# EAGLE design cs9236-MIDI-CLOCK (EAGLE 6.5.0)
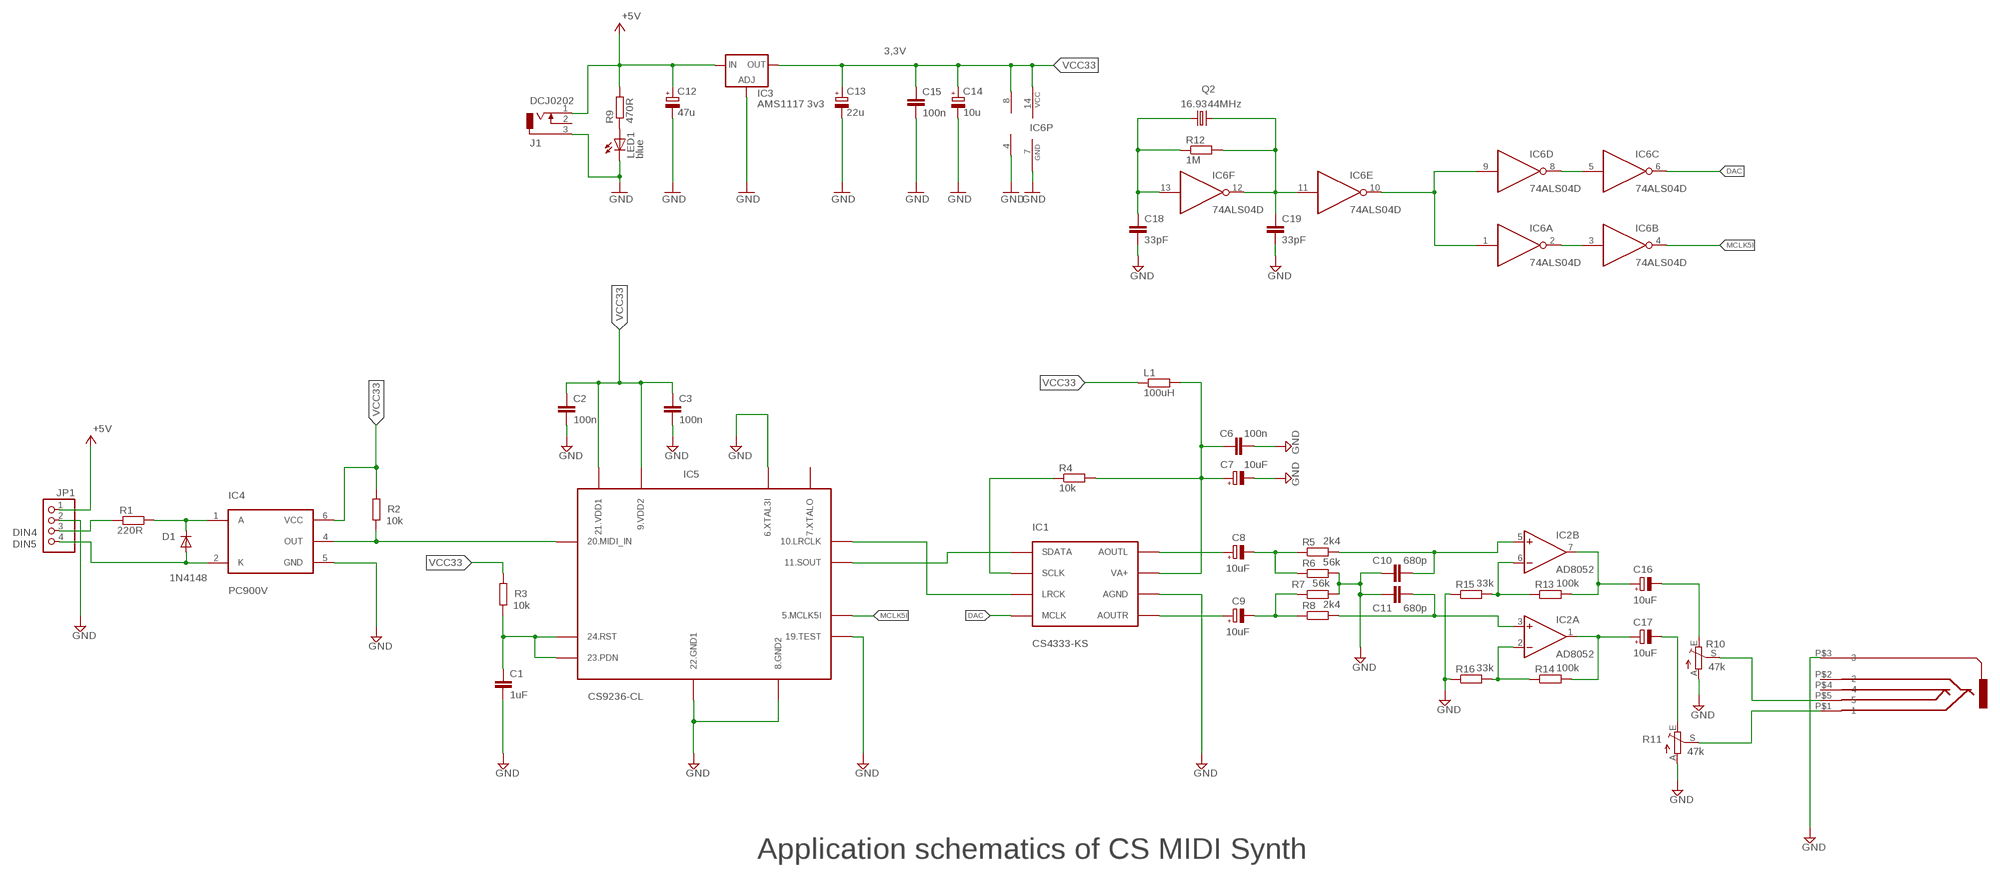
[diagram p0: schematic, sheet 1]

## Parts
C1  1uF  C-EUC0805  [C0805]
C2  100n  C-EUC0805  [C0805]
C3  100n  C-EUC0805  [C0805]
C6  100n  C-EUC0805  [C0805]
C7  10uF  CPOL-EUSMCC  [SMC_C]
C8  10uF  CPOL-EUSMCC  [SMC_C]
C9  10uF  CPOL-EUSMCC  [SMC_C]
C10  680p  C-EUC0805  [C0805]
C11  680p  C-EUC0805  [C0805]
C12  47u  CPOL-EUSMCD  [SMC_D]
C13  22u  CPOL-EUSMCD  [SMC_D]
C14  10u  CPOL-EUSMCB  [SMC_B]
C15  100n  C-EUC0805  [C0805]
C16  10uF  CPOL-EUSMCC  [SMC_C]
C17  10uF  CPOL-EUSMCC  [SMC_C]
C18  33pF  C-EUC0805  [C0805]
C19  33pF  C-EUC0805  [C0805]
D1  1N4148  1N4148DO35-7  [DO35-7]
IC1  CS4333-KS  [SO8]
IC2  AD8052  LM1458D  [SO08]
IC3  AMS1117 3v3  LD117AS33TR  [SOT223]
IC4  PC900V  [DIP6STD]
IC5  CS9236-CL  [PLCC28]
IC6  74ALS04D  [SO14]
J1  DCJ0202  [DCJ0202]
JP1  PINHD-1X4  [1X04]
L1  100uH  R-EU_0207/10  [0207/10]
LED1  blue  LEDSML0805  [SML0805]
Q2  16.9344MHz  CRYSTALHC49UP  [HC49UP]
R1  220R  R-EU_R0805  [R0805]
R2  10k  R-EU_R0805  [R0805]
R3  10k  R-EU_R0805  [R0805]
R4  10k  R-EU_R0805  [R0805]
R5  2k4  R-EU_R0805  [R0805]
R6  56k  R-EU_R0805  [R0805]
R7  56k  R-EU_R0805  [R0805]
R8  2k4  R-EU_R0805  [R0805]
R9  470R  R-EU_R0805  [R0805]
R10  47k  TRIM_EU-CT6  [CT6]
R11  47k  TRIM_EU-CT6  [CT6]
R12  1M  R-EU_R0805  [R0805]
R13  100k  R-EU_R0805  [R0805]
R14  100k  R-EU_R0805  [R0805]
R15  33k  R-EU_R0805  [R0805]
R16  33k  R-EU_R0805  [R0805]
U$3  JACK3.5  [JACK3.5]

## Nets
+5V: C12.+ IC3.3(IN) J1.1 JP1.1 R9.2
DAC: IC1.4(MCLK) IC6.6(C:O)
GND: C1.2 C2.2 C3.2 C6.2 C7.- C10.1 C11.1 C12.- C13.- C14.- C15.2 C18.2 C19.2 IC1.6(AGND) IC2.4(P:V-) IC3.1(ADJ) IC4.5(GND) IC5.6(6.XTAL3I) IC5.8(8.GND2) IC5.19(19.TEST) IC5.22(22.GND1) IC6.7(P:GND) J1.3 JP1.2 LED1.C R6.2 R7.2 R10.A R11.A R15.1 R16.1 U$3.P$3
MCLK5I: IC5.5(5.MCLK5I) IC6.4(B:O)
N$1: IC2.6(B:-IN) R13.1 R15.2
N$2: IC1.3(LRCK) IC5.10(10.LRCLK)
N$3: IC1.1(SDATA) IC5.11(11.SOUT)
N$4: C1.1 IC5.23(23.PDN) IC5.24(24.RST) R3.1
N$5: D1.C IC4.1(A) R1.1
N$6: IC4.4(OUT) IC5.20(20.MIDI_IN) R2.1
N$7: C9.+ IC1.5(AOUTR)
N$8: C8.+ IC1.8(AOUTL)
N$9: C6.1 C7.+ IC1.7(VA+) L1.2 R4.2
N$10: IC1.2(SCLK) R4.1
N$11: C8.- R5.1 R6.1
N$12: C9.- R7.1 R8.1
N$13: D1.A IC4.2(K) JP1.4
N$14: C18.1 IC6.13(F:I) Q2.1 R12.1
N$15: C11.2 IC2.3(A:+IN) R8.2
N$16: C10.2 IC2.5(B:+IN) R5.2
N$17: IC2.2(A:-IN) R14.1 R16.2
N$18: LED1.A R9.1
N$19: C16.+ IC2.7(B:OUT) R13.2
N$20: C17.+ IC2.1(A:OUT) R14.2
N$21: C16.- R10.E
N$22: C17.- R11.E
N$23: JP1.3 R1.2
N$24: R10.S U$3.P$5
N$25: R11.S U$3.P$1
N$26: C19.1 IC6.11(E:I) IC6.12(F:O) Q2.2 R12.2
N$27: IC6.1(A:I) IC6.9(D:I) IC6.10(E:O)
N$28: IC6.2(A:O) IC6.3(B:I)
N$29: IC6.5(C:I) IC6.8(D:O)
VCC33: C2.1 C3.1 C13.+ C14.+ C15.1 IC2.8(P:V+) IC3.4(OUT) IC4.6(VCC) IC5.9(9.VDD2) IC5.21(21.VDD1) IC6.14(P:VCC) L1.1 R2.2 R3.2
Unconnected: IC5.7(7.XTALO) J1.2 U$3.P$2 U$3.P$4

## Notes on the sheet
- 3,3V
- DIN4
- DIN5
- Application schematics of CS MIDI Synth

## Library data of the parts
C1-C3 C6 C10 C11 C15 C18 C19 = rcl:C-EU: CAPACITOR, European symbol
C7-C9 C12-C14 C16 C17 = rcl:CPOL-EU: POLARIZED CAPACITOR, European symbol
D1 = diode:1N4148: DIODE
IC1 = crystal-midi:CS4333-KS
IC2 = linear:*1458: OP AMP
IC3 = v-reg:LD117A?*: Low drop fixed and adjustable positive voltage regulators 1 A Source: http://www.st.com/stonline/products/literature/ds/7194/ld1117axx.pdf
IC4 = pc900:PC900V
IC5 = crystal-midi:CS9236-CL
IC6 = 74xx-us:74*04: Hex INVERTER
J1 = con-jack:DCJ0202: DC POWER JACK Source: DCJ0202.pdf; OC_FARNELL: unknown; OC_NEWARK: unknown
JP1 = pinhead:PINHD-1X4: PIN HEADER
L1 R1-R9 R12-R16 = rcl:R-EU_: RESISTOR, European symbol
LED1 = led:LED: LED
Q2 = crystal:CRYSTAL: CRYSTAL; OC_FARNELL: unknown; OC_NEWARK: unknown
R10 R11 = pot:TRIM_EU-: POTENTIOMETER
U$3 = CART-Z7:JACK3.5

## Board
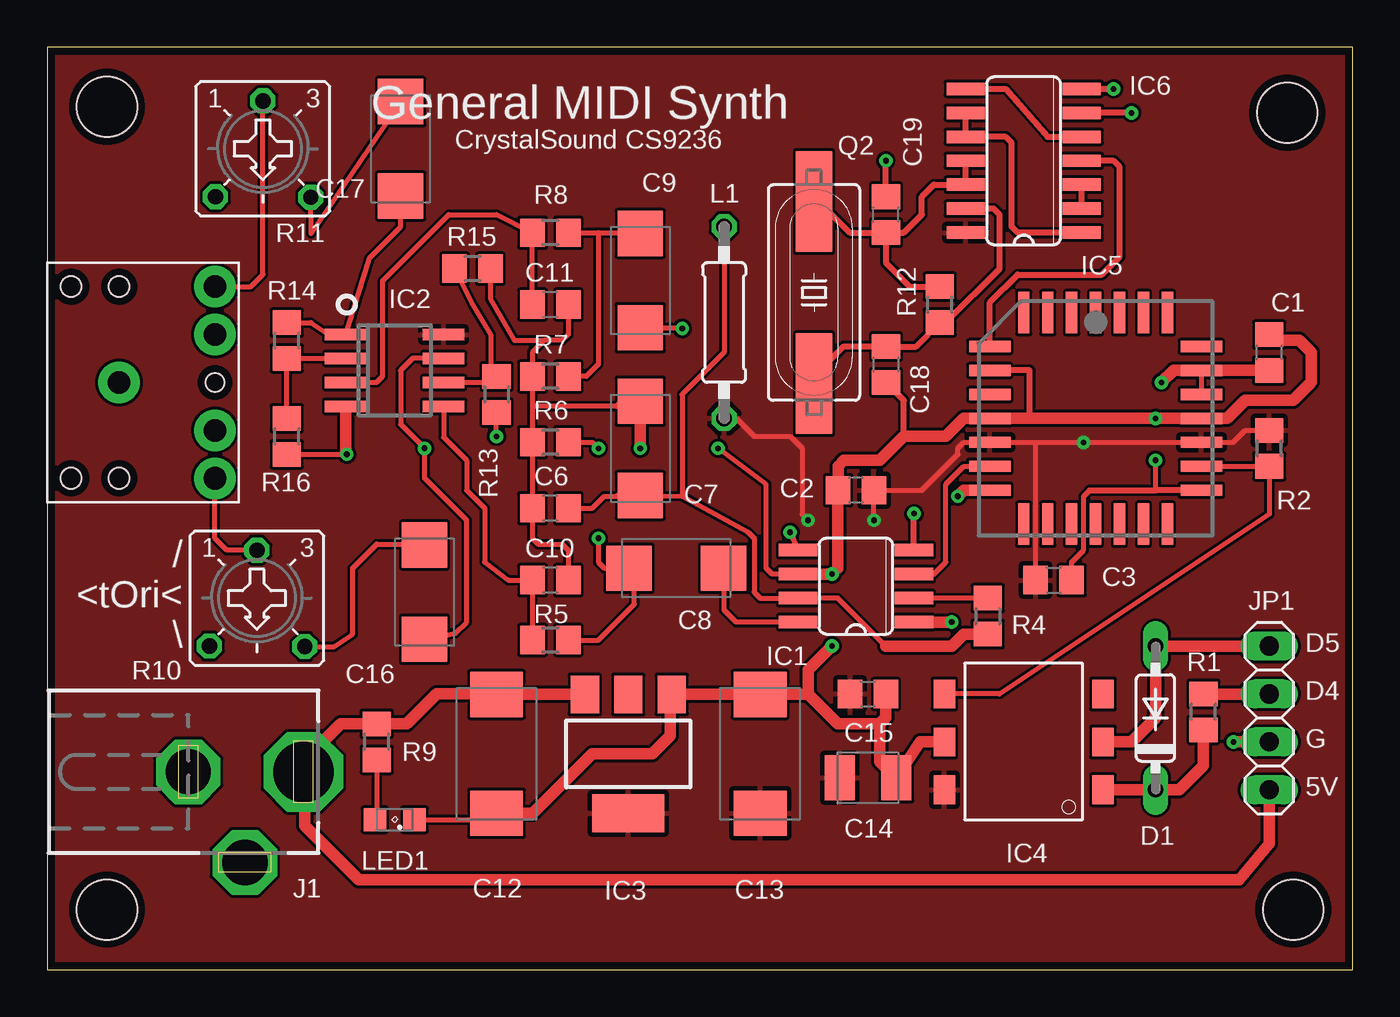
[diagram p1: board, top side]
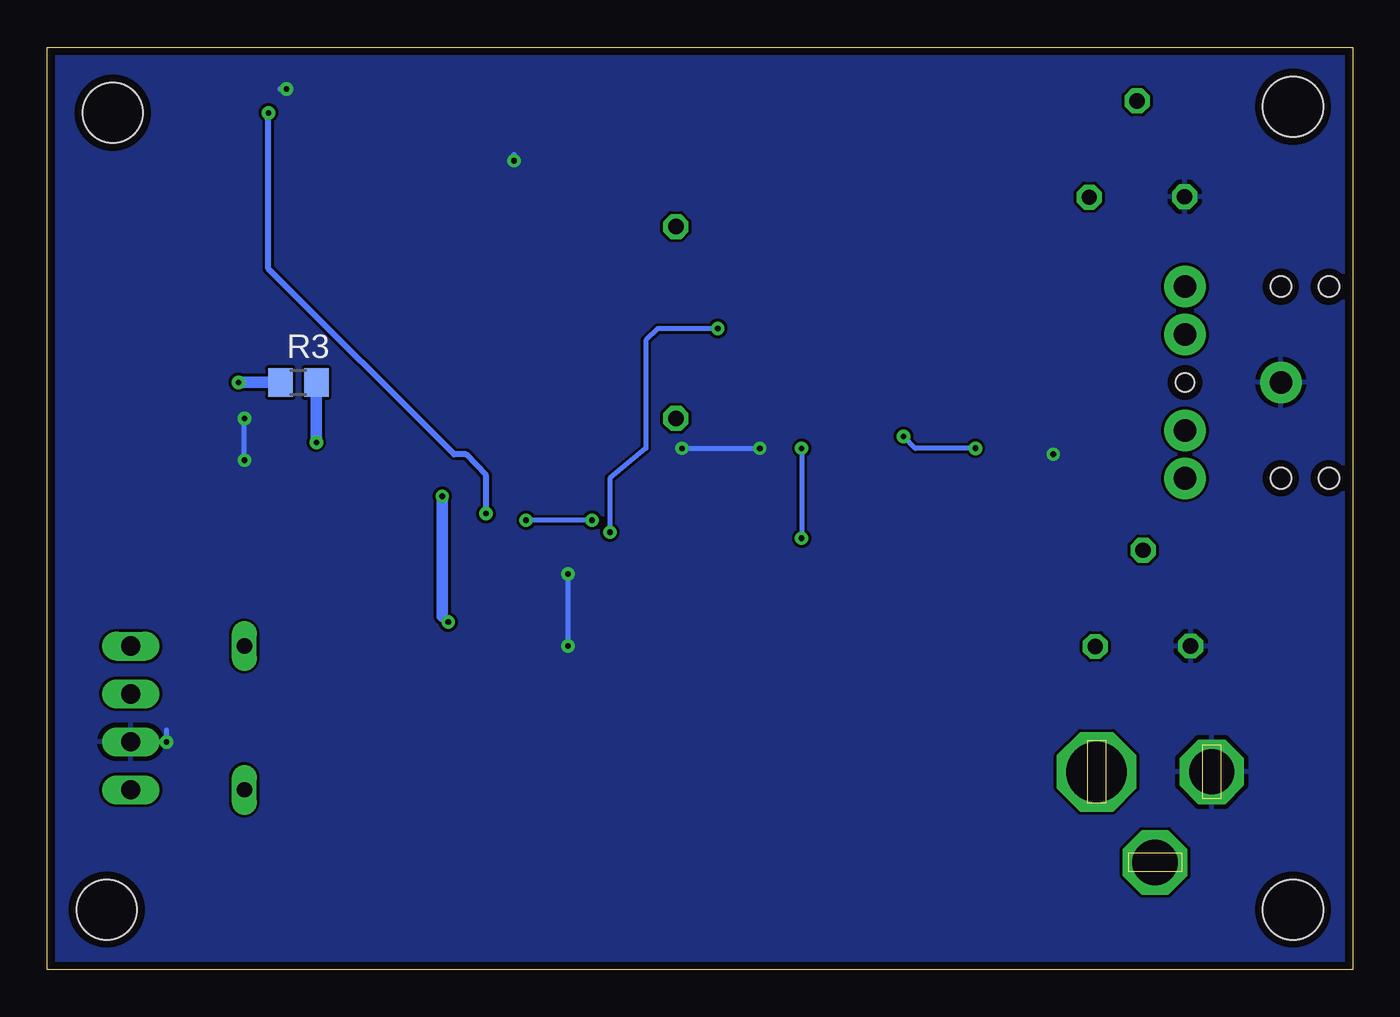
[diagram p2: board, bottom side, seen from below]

Size 69.2 x 48.88 mm. Coordinates in mm from the lower left corner, seen from the top.
Outline: 0,0 69.2,0 69.2,48.88 0,48.88 0,0
Copper layers (1*16): Top 0.035mm / dielectric 1.5mm / Bottom 0.035mm
Design rules "default": minimum track width 5mil, minimum drill 8mil, track to track 6mil, track to pad 6mil, pad to pad 6mil, via to via 6mil, smd to smd 6mil, copper to edge 16mil, drill to drill 8mil, minimum pad ring 10mil, minimum via ring 8mil, stop-mask expansion 4mil, vias tented up to drill 0mil, thermal gap 10mil
Holes 3.2 mm at 3.17,45.72 65.72,45.4 66.04,3.18 3.17,3.18

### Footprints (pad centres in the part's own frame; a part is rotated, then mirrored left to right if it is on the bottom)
C0805 = smd 1.3 x 1.5: 1 -0.95,0; 2 0.95,0
SMC_C = smd 2.4 x 2.4: + -2.5,0; - 2.5,0
SMC_D = smd 2.4 x 2.8: + -3.15,0; - 3.15,0
SMC_B = smd 1.6 x 2.4: + -1.5,0; - 1.5,0
DO35-7 = drill 0.813 long: A 3.81,0; C -3.81,0
SO8 = smd 0.66 x 2.032: 1 -1.905,-3.073; 2 -0.635,-3.073; 3 0.635,-3.073; 4 1.905,-3.073; 5 1.905,3.073; 6 0.635,3.073; 7 -0.635,3.073; 8 -1.905,3.073
SO08 = smd 0.6 x 2.2: 1 -1.905,-2.6; 2 -0.635,-2.6; 3 0.635,-2.6; 4 1.905,-2.6; 5 1.905,2.6; 6 0.635,2.6; 7 -0.635,2.6; 8 -1.905,2.6
SOT223 = smd 1.5 x 2: 1 -2.3,-3.15; 2 0,-3.15; 3 2.3,-3.15 | smd 3.8 x 2: 4 0,3.15
DIP6STD = smd 1.524 x 1.143: 1 -2.54,-4.204; 2 0,-4.204; 3 2.54,-4.204; 4 2.54,4.204; 5 0,4.204; 6 -2.54,4.204
PLCC28 = smd 0.6 x 2.2: 1 0,5.6; 2 -1.27,5.6; 3 -2.54,5.6; 4 -3.81,5.6; 12 -3.81,-5.6; 13 -2.54,-5.6; 14 -1.27,-5.6; 15 0,-5.6; 16 1.27,-5.6; 17 2.54,-5.6; 18 3.81,-5.6; 26 3.81,5.6; 27 2.54,5.6; 28 1.27,5.6 | smd 2.2 x 0.6: 5 -5.6,3.81; 6 -5.6,2.54; 7 -5.6,1.27; 8 -5.6,0; 9 -5.6,-1.27; 10 -5.6,-2.54; 11 -5.6,-3.81; 19 5.6,-3.81; 20 5.6,-2.54; 21 5.6,-1.27; 22 5.6,0; 23 5.6,1.27; 24 5.6,2.54; 25 5.6,3.81
SO14 = smd 0.66 x 2.032: 1 -3.81,-3.073; 2 -2.54,-3.073; 3 -1.27,-3.073; 4 0,-3.073; 5 1.27,-3.073; 6 2.54,-3.073; 7 3.81,-3.073; 8 3.81,3.073; 9 2.54,3.073; 10 1.27,3.073; 11 0,3.073; 12 -1.27,3.073; 13 -2.54,3.073; 14 -3.81,3.073
DCJ0202 = drill 3.2 pad 4 octagon: 1 0,3.1 | drill 2.4 pad 3.2 octagon: 2 4.8,0; 3 0,-3
1X04 = drill 1.016 long: 1 -3.81,0; 2 -1.27,0; 3 1.27,0; 4 3.81,0
0207/10 = drill 0.813 octagon: 1 -5.08,0; 2 5.08,0
SML0805 = smd 1.2 x 1.2: A 1.05,0; C -1.05,0
HC49UP = smd 5.334 x 1.93: 1 -4.826,0; 2 4.826,0
R0805 = smd 1.3 x 1.5: 1 -0.95,0; 2 0.95,0
CT6 = drill 0.813 octagon: A 2.515,2.54; E -2.54,2.565; S 0,-2.54
JACK3.5 = drill 1.2 pad 2.2: P$1 0,5.08; P$2 0,2.54; P$3 -5.08,0; P$4 0,-2.54; P$5 0,-5.08 | hole 1: 0,0 | hole 1.1: -5.08,-5.08; -5.08,5.08; -7.62,5.08; -7.62,-5.08

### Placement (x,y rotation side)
C1  64.77,32.7 90 top
C2  42.86,25.4 180 top
C3  53.34,20.64 0 top
C6  26.67,24.45 180 top
C7  31.43,27.62 90 top
C8  33.34,21.27 180 top
C9  31.43,36.51 90 top
C10  26.67,20.64 180 top
C11  26.67,35.24 180 top
C12  23.81,11.43 270 top
C13  37.78,11.43 90 top
C14  43.5,10.16 0 top
C15  43.5,14.61 0 top
C16  20,20 90 top
C17  18.73,43.5 90 top
C18  44.45,32.07 270 top
C19  44.45,40 90 top
D1  58.74,13.34 90 top
IC1  42.86,20.32 90 top
IC2  18.41,31.75 270 top
IC3  30.8,11.43 180 top
IC4  51.75,12.07 90 top
IC5  55.56,29.21 0 top
IC6  51.75,42.86 90 top
J1  10.48,10.48 270 top
JP1  64.77,13.34 90 top
L1  35.88,34.29 90 top
LED1  18.41,7.94 180 top
Q2  40.64,35.88 90 top
R1  61.28,13.65 90 top
R2  64.77,27.62 90 top
R3  55.88,31.11 0 bottom
R4  49.85,18.73 270 top
R5  26.67,17.46 180 top
R6  26.67,27.94 180 top
R7  26.67,31.43 180 top
R8  26.67,39.05 180 top
R9  17.46,12.07 90 top
R10  11.11,19.68 180 top
R11  11.43,43.5 180 top
R12  47.31,35.24 90 top
R13  23.81,30.48 270 top
R14  12.7,33.34 90 top
R15  22.54,37.15 180 top
R16  12.7,28.26 90 top
U$3  8.89,31.11 0 top

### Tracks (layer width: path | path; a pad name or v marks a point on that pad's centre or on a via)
+5V
  Top 0.254: 22.86,14.9 C12.+ 23.15,14.61
  Top 0.61: 23.15,14.61 20.64,14.61 19.05,13.02 R9.2 15.56,13.02 13.65,11.11 13.65,10.55 | C12.+ IC3.3 | JP1.1 64.77,6.67 63.18,4.76 16.51,4.76 13.65,7.62 13.65,10.55 | 13.65,10.55 J1.1
DAC  (via drill 0.3)
  Top 0.305: IC1.4 v45.94,24.16 | v57.47,45.4 IC6.6
  Bottom 0.305: v45.94,24.16 45.94,26.19 46.99,27.31 47.62,27.31 57.47,37.15 v57.47,45.4
GND  (via drill 0.3, 0.3 pad 0.6)
  Top 0.254: C3.2 54.29,21.59 54.93,22.22 54.93,25.08 55.25,25.4 | 58.74,25.4 v58.74,26.99 | 65.4,33.34 C1.2 | v41.59,20.96 41.91,21.27 | IC1.6 38.42,20.96 38.1,21.27 38.1,25.72 v35.56,27.62 | C11.1 27.62,33.65 27.3,33.34 26.35,33.34 | 26.35,33.34 25.72,32.7 R7.2 25.72,29.85 | 25.72,29.85 R6.2 C6.2 25.72,23.49 25.72,22.86 26.04,22.54 27.3,22.54 27.62,22.22 27.62,21.28 C10.1 | C7.- 30.44,30.12 30.16,29.85 25.72,29.85 | C2.2 | LED1.C 22.83,7.94 C12.- | 33.02,14.5 IC3.1 | C15.2 | R16.1 v15.87,27.31 | R15.1 23.49,35.56 24.76,33.34 26.35,33.34
  Top 0.305: 55.25,25.4 58.74,25.4 IC5.19 | IC5.8 52.07,29.21 52.07,31.75 IC5.6 | 45.4,28.26 45.4,30.17 C18.2 | C19.2 v44.45,42.86 | IC6.7 v56.51,46.67
  Top 0.61: 46.67,28.26 47.62,28.26 48.58,29.21 IC5.8 v58.74,29.21 IC5.22 62.55,29.21 63.5,30.16 66.04,30.16 66.99,31.11 66.99,32.7 66.36,33.34 65.4,33.34 | C2.2 41.91,26.67 42.23,26.99 44.13,26.99 45.4,28.26 46.67,28.26 | IC1.6 v41.59,20.96 | v31.43,27.62 C7.- | 41.91,21.27 C2.2 | C12.- 25.74,8.28 28.89,11.43 32.07,11.43 33.02,12.38 33.02,14.5 | IC3.1 C13.- 40.35,14.58 | 40.35,14.58 41.91,13.02 44.13,13.02 | 44.13,13.02 44.45,13.34 C15.2 | 44.13,13.02 44.13,11.02 C14.- 46.28,12.07 IC4.5 | 40.35,14.58 40.35,15.9 v41.59,17.14 | JP1.2 v62.87,12.07 | IC2.4 15.82,27.36 v15.87,27.31
  Bottom 0.254: v58.74,26.99 v58.74,29.21 | v35.56,27.62 v31.43,27.62 | v41.59,17.14 v41.59,20.96 | v62.87,12.07 62.87,12.7
  Bottom 0.305: v44.45,42.86 44.45,43.18 | v56.51,46.67 56.83,46.67
  pour Bottom: 0.32,48.58 68.9,48.58 68.9,0.32 0.32,0.32
MCLK5I
  Top 0.305: IC5.5 49.96,35.36 51.44,36.83 55.88,36.83 56.83,37.78 56.83,42.54 56.51,42.86 IC6.4
N$1
  Top 0.254: IC2.6 23.5,31.11 R13.1 23.5,31.75 23.5,33.65 22.54,35.24 R15.2
N$2
  Top 0.254: IC1.3 46.99,20.96 47.62,21.59 47.62,25.72 48.58,26.67 IC5.10
N$3  (via drill 0.3 pad 0.6)
  Top 0.61: IC1.1 v47.94,18.42 | v48.26,25.08 48.58,25.4 IC5.11
  Bottom 0.254: v47.94,18.42 48.26,18.73
  Bottom 0.61: 48.26,18.73 v48.26,25.08
N$4  (via drill 0.3 pad 0.6)
  Top 0.254: IC5.24 IC5.23
  Top 0.61: C1.1 IC5.24 59.69,31.75 v59.06,31.11
  Bottom 0.61: v59.06,31.11 R3.1
N$5
  Top 0.61: R1.1 61.28,10.79 60.01,9.52 D1.C IC4.1
N$6
  Top 0.254: R2.1 IC5.20 R2.1 64.77,24.13 50.48,14.61 IC4.4
N$7  (via drill 0.3 pad 0.6)
  Top 0.254: C9.+ 33.61,34.01 v33.65,33.97 | v39.37,23.18 IC1.5
  Bottom 0.254: v33.65,33.97 36.83,33.97 37.47,33.34 37.47,27.62 39.37,26.04 v39.37,23.18
N$8
  Top 0.254: IC1.8 36.51,18.42 35.88,19.05 35.88,21.23 C8.+
N$9
  Top 0.254: 44.45,17.14 41.91,19.68 IC1.7 37.78,19.68 37.47,20 37.47,22.86 37.15,23.18 33.65,25.08 | L1.2 35.88,32.7 33.65,30.48 33.65,25.08 | 33.65,25.08 30.2,25.12 C7.+ 31.08,25.08 29.53,25.08 28.89,24.45 C6.1
  Top 0.61: R4.2 48.58,17.78 47.94,17.14 44.45,17.14
N$10
  Top 0.254: R4.1 IC1.2
N$11  (via drill 0.3 pad 0.6)
  Top 0.254: R5.1 29.21,17.46 31.11,19.37 31.11,21.23 C8.- 29.53,21.27 29.21,21.59 v29.21,22.86 | R6.1 28.89,27.94 v29.21,27.62
  Bottom 0.254: v29.21,27.62 v29.21,22.86
N$12
  Top 0.254: 29.21,39.05 31.08,39.05 C9.- | R8.1 29.21,39.05 | 29.21,39.05 29.21,32.07 28.58,31.43 R7.1
N$13
  Top 0.61: IC4.2 57.47,12.07 58.74,13.34 D1.A JP1.4
N$14
  Top 0.305: Q2.1 40.64,31.43 42.23,33.02 C18.1 46.03,33.02 R12.1 47.63,34.29 50.48,37.15 50.48,40 50.17,40.32 IC6.13
N$15
  Top 0.254: IC2.3 17.46,31.11 17.78,31.43 17.78,36.51 21.27,40 23.82,40 R8.2 C11.2
N$16
  Top 0.254: R5.2 C10.2 24.45,20.64 23.18,21.59 23.18,24.45 22.22,25.4 22.22,26.99 21.01,28.2 IC2.5
N$17
  Top 0.254: R16.2 R14.1 13.97,32.39 14.29,32.39 IC2.2
N$18
  Top 0.254: R9.1 17.46,8.04 LED1.A
N$19  (via drill 0.3 pad 0.13)
  Top 0.254: C16.+ 21.63,17.82 22.22,18.42 22.22,23.81 20,26.04 v20,27.62 18.73,28.89 18.73,31.75 19.37,32.39 IC2.7 | v23.81,28.26 R13.2
  Bottom 0.254: v20,27.62 23.18,27.62 v23.81,28.26
N$20
  Top 0.254: C17.+ 18.73,39.37 17.08,37.72 IC2.1 14.92,33.65 13.97,34.29 R14.2
N$21
  Top 0.254: R10.E 15.21,17.12 16.19,17.78 16.19,21.27 17.46,22.54 19.72,22.54 C16.-
N$22
  Top 0.254: C17.- 13.98,39.01 R11.E
N$23
  Top 0.254: 65.09,14.6 JP1.3
  Top 0.61: R1.2 65.09,14.6
N$24
  Top 0.254: R10.S 9.52,22.22 8.89,22.86 U$3.P$5
N$25
  Top 0.254: U$3.P$1 10.79,36.19 11.43,36.83 R11.S
N$26
  Top 0.305: Q2.2 40.89,40.7 42.54,39.05 C19.1 | C19.1 44.45,37.46 45.72,36.19 R12.2 | C19.1 45.4,39.06 46.36,40 46.36,40.96 46.99,41.59 IC6.12 IC6.11
N$27
  Top 0.305: IC6.1 51.44,39.05 51.12,39.37 51.12,43.82 50.8,44.13 IC6.10 IC6.9
N$28
  Top 0.305: IC6.2 IC6.3
N$29
  Top 0.305: IC6.8 50.8,46.67 53.02,44.13 IC6.5
VCC33  (via drill 0.3 pad 0.6)
  Top 0.254: 52.39,27.94 IC5.9 48.58,27.94 48.26,27.62 48.26,27.31 46.36,25.4 C2.1 v43.82,23.81 | 52.39,27.94 v54.93,27.94 IC5.21 62.87,27.94 63.5,28.57 R2.2 | C3.1 52.39,27.94 | L1.1 36.51,29.21 37.47,28.26 39.37,28.26 40.01,27.62 40.01,24.13 v40.32,23.81
  Bottom 0.254: v54.93,27.94 | v40.32,23.81 v43.82,23.81
  Bottom 0.61: R3.2 v54.93,27.94
  pour Top: 0.32,48.58 68.9,48.58 68.9,0.32 0.32,0.32

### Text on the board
tNames: General MIDI Synth | CrystalSound CS9236 | / / <tOri< / \\ | D5 | D4 | G | 5V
